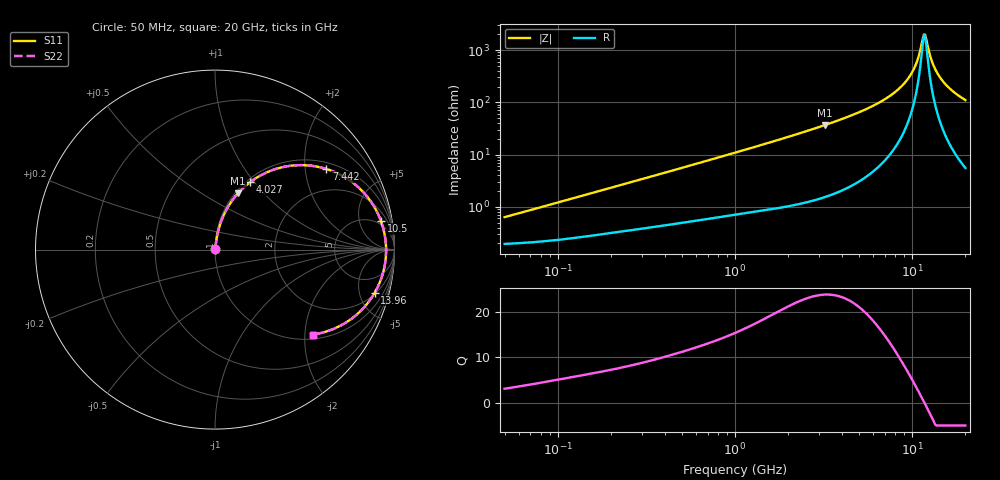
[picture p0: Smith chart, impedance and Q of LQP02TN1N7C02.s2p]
!Murata Part Number: LQP02TN1N7C02
!These Parameters are Measured in Series Mode Connection
!  o--[Z]--o
!Port1  Port2
!  o-------o
!Freq. Start=50[MHz] Stop=20[GHz], 401[Steps]
# Hz S RI R 50
!Freq.(Hz) S11(Real) S11(Imag) S21(Real) S21(Imag) S12(Real) S12(Imag) S22(Real) S22(Imag)
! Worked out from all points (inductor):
!   401 points, 50 MHz to 20 GHz, reference 50 ohm
!   read as one part in series: L = 1.91 nH near 51.52 MHz
!   highest Q = 23.9 at 3.217 GHz (marker M1), where L = 1.81 nH
!   self-resonance near 11.75 GHz
!   S11 on the Smith chart (normalised r, x): 50 MHz: 1.00, +0.01; 4.027 GHz: 1.04, +0.96; 7.442 GHz: 1.19, +2.60; 10.5 GHz: 4, +10; 13.96 GHz: 2.16, -6.90; 20 GHz: 1.11, -2.20
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5e7  0.00198 0.00601  0.998 -0.00601  0.998 -0.00601  0.00198 0.00601
1.364002e8  0.00289 0.0159  0.9971 -0.0159  0.9971 -0.0159  0.00289 0.0159
3.721004e8  0.00593 0.0411  0.9941 -0.0411  0.9941 -0.0411  0.00593 0.0411
1e9  0.0183 0.1055  0.9817 -0.1055  0.9817 -0.1055  0.0183 0.1055
2.728004e9  0.0942 0.2716  0.9058 -0.2716  0.9058 -0.2716  0.0942 0.2716
3.216634e9  0.1282 0.314  0.8718 -0.314  0.8718 -0.314  0.1282 0.314
4.026975e9  0.1971 0.377  0.8029 -0.377  0.8029 -0.377  0.1971 0.377
5.515528e9  0.362 0.4559  0.638 -0.4559  0.638 -0.4559  0.362 0.4559
7.442007e9  0.6203 0.4494  0.3797 -0.4494  0.3797 -0.4494  0.6203 0.4494
8.389408e9  0.742 0.3914  0.258 -0.3914  0.258 -0.3914  0.742 0.3914
9.178299e9  0.828 0.3179  0.172 -0.3179  0.172 -0.3179  0.828 0.3179
9.892087e9  0.8883 0.2365  0.1117 -0.2365  0.1117 -0.2365  0.8883 0.2365
1.050288e10  0.9244 0.1599  0.0756 -0.1599  0.0756 -0.1599  0.9244 0.1599
1.082228e10  0.9374 0.1186  0.0626 -0.1186  0.0626 -0.1186  0.9374 0.1186
1.149051e10  0.952 0.0322  0.048 -0.0322  0.048 -0.0322  0.952 0.0322
1.183995e10  0.9532 -0.0119  0.0468 0.0119  0.0468 0.0119  0.9532 -0.0119
1.201863e10  0.9523 -0.034  0.0477 0.034  0.0477 0.034  0.9523 -0.034
1.295331e10  0.9326 -0.1417  0.0674 0.1417  0.0674 0.1417  0.9326 -0.1417
1.396067e10  0.8902 -0.2396  0.1098 0.2396  0.1098 0.2396  0.8902 -0.2396
1.504638e10  0.8302 -0.3222  0.1698 0.3222  0.1698 0.3222  0.8302 -0.3222
1.621653e10  0.7589 -0.3864  0.2411 0.3864  0.2411 0.3864  0.7589 -0.3864
2e10  0.5465 -0.4734  0.4535 0.4734  0.4535 0.4734  0.5465 -0.4734
